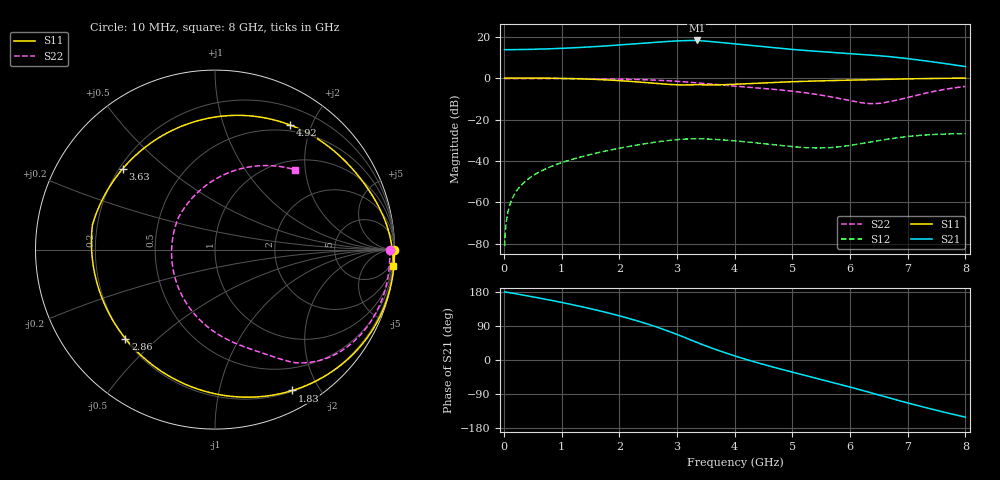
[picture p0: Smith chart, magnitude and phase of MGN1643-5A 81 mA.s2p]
! Port[1] = GATE
! Port[2] = DRAIN
! [Type]  S-parameter s2p file touchstone ver. 1.0
! [Object]  MGN1643-5A
! [Bias]  81 mA
! [Version]  1.0
! [Date]  Thu May 19 10:51:16 2026
! [Source]  This file was created in JSC "ICC Milandr".
! [Disclaimer] Property of JSC "ICC Milandr". Unauthorized reproduction and/or distribution is strictly prohibited.
!  The file and the data are provided "AS IS" and with all faults and disclaim all warranties, express and implied, including
!  without limitation any implied warranties of merchantability, fitness for a particular purpose.
!  JSC "ICC Milandr" assumes no liability for:
!  1) the accuracy of the data provided;
!  2) the proper functioning of this data;
!  3) infringement of patents, copyrights or intellectual property rights resulting from the use of this data.
!  JSC "ICC Milandr" reserves the right to make changes to the products and the data without prior notice.
!  Please, be aware that your receipt and use of the file provided shall serve as acceptance of these terms and conditions.
!  If you do not accept these terms, you should return or destroy this file and any other accompanying information immediately.
# Hz S MA R 12.5
! freq  S11mag  S11ang  S21mag  S21ang  S12mag  S12ang  S22mag  S22ang
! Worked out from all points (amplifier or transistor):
!   800 points, 10 MHz to 8 GHz, reference 12.5 ohm
!   highest |S21| = 18.2 dB at 3.34 GHz (marker M1)
!   |S21| within 3 dB of that: 1.56 GHz to 4.477 GHz (2.917 GHz wide, 96.6 % of centre)
!   unconditionally stable (mu >= 1): 4.909 GHz to 5.594 GHz
!   at 1.34 GHz: K = 0.23, MSG = 26.4 dB, |S12| = -38.0 dB
!   at 4.01 GHz: K = 0.73, MSG = 23.4 dB, |S12| = -30.3 dB
!   at 8 GHz: K = 0.23, MSG = 16.2 dB, |S12| = -26.9 dB
!   S11 on the Smith chart (normalised r, x): 10 MHz: open; 1.83 GHz: 0.21, -1.67; 2.86 GHz: 0.20, -0.40; 3.63 GHz: 0.21, +0.36; 4.92 GHz: 0.42, +1.69; 8 GHz: 1, -22
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1e7  1 -0.2  4.849 179.7  8.768e-05 86.4  0.9733 -0.1
1.1e8  1.001 -3.0  4.853 177.2  0.0009555 87.4  0.9741 -1.4
3.1e8  1.001 -8.6  4.889 171.9  0.002705 83.6  0.9753 -4.1
8.9e8  0.9873 -25.6  5.148 155.3  0.008031 71.0  0.9749 -12.0
1.35e9  0.9553 -41.2  5.511 140.5  0.0127 59.5  0.9682 -18.6
1.83e9  0.8958 -61.2  6.053 123.3  0.01817 45.8  0.9524 -26.1
2.27e9  0.8166 -85.6  6.708 105.1  0.02377 30.8  0.926 -33.8
2.68e9  0.7333 -117.5  7.403 85.3  0.02916 14.0  0.8844 -41.7
2.86e9  0.7035 -135.2  7.688 75.5  0.03129 5.5  0.8589 -45.4
3.1e9  0.6836 -162.3  7.977 61.4  0.0335 -6.9  0.817 -50.3
3.34e9  0.6967 168.6  8.089 46.5  0.03451 -20.2  0.7683 -55.0
3.48e9  0.6855 153.8  7.829 38.3  0.03407 -26.9  0.7379 -57.2
3.63e9  0.6836 138.8  7.515 29.9  0.03331 -33.5  0.7073 -59.3
3.81e9  0.6919 122.5  7.114 20.3  0.0321 -40.4  0.6736 -61.9
4.01e9  0.71 106.6  6.667 10.3  0.0305 -46.9  0.6394 -64.9
4.44e9  0.7594 80.1  5.794 -9.2  0.0267 -56.1  0.5722 -72.4
4.92e9  0.8101 59.1  5.022 -28.9  0.02274 -57.6  0.4956 -83.8
5.34e9  0.8457 45.4  4.507 -45.3  0.02067 -50.3  0.4189 -98.2
6.02e9  0.8931 28.8  3.872 -72.2  0.02399 -31.1  0.2811 -140.1
6.67e9  0.9378 16.1  3.314 -100.0  0.03379 -26.9  0.2692 140.1
7.3e9  0.9729 5.9  2.608 -125.2  0.04229 -44.1  0.4297 81.1
8e9  0.9969 -5.2  1.898 -150.7  0.04542 -63.8  0.6296 44.9
